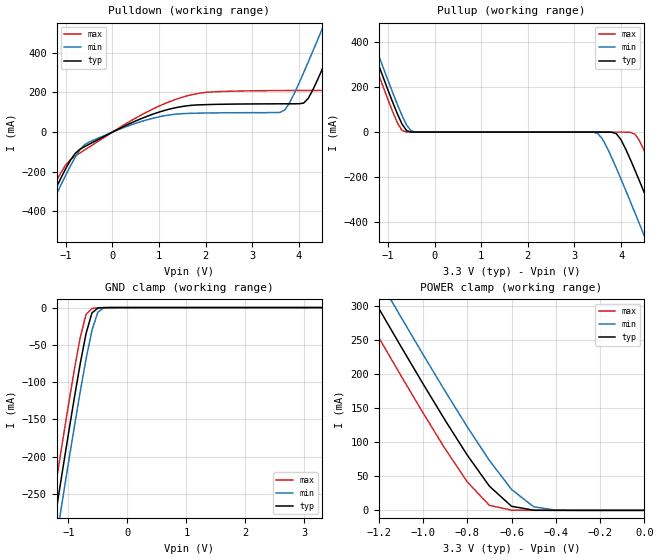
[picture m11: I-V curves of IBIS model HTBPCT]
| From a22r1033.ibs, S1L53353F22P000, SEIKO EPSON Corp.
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[Model]   HTBPCT
Model_type   Output
Polarity   Non-Inverting
|   typ   min   max
C_comp   5.0pF   4.0pF   6.0pF
|   typ   min   max
[Voltage range]   3.3   3.0   3.6
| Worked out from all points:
|   slope of the pulldown table from 0 to 0.495 V, typ, clamps not added: 8.88 ohm
|   GND clamp passes 1 mA (typ) near -0.51 V on its own axis
|   POWER clamp passes 1 mA (typ) near -0.51 V on its own axis
[Pulldown]
|   Voltage   I(typ)   I(min)   I(max)
-3.3V     -1.365A    -1.401A    -1.33A
-1.7V     -529.5mA   -566.9mA   -493.2mA
-1.1V     -229.2mA   -264.4mA   -201.9mA
-800mV    -107.9mA   -126.6mA   -121mA
200mV     23.74mA    19.01mA    29.63mA
1.7V      135.1mA    94.74mA    188.4mA
3.7V      142.6mA    112.5mA    209.5mA
4.1V      146mA      298.6mA    209.8mA
4.5V      316.8mA    521mA      210.2mA
4.9V      540.2mA    749.4mA    339.3mA
5.3V      769.7mA    980.3mA    562.8mA
6.6V      1.527A     1.738A     1.318A
[Pullup]
|   Voltage   I(typ)   I(min)   I(max)
-3.3V     1.514A     1.553A     1.476A
-1.6V     524.3mA    566.8mA    482.3mA
-1.5V     467mA      509.6mA    424.7mA
-800mV    81.11mA    122.6mA    41.82mA
-600mV    5.969mA    30.7mA     281.7uA
3.5V      -273.4nA   -6.157mA   -6.736nA
3.9V      -7.117mA   -160.6mA   -899.7nA
4.3V      -170mA     -359.4mA   -9.189mA
4.5V      -269.6mA   -461.5mA   -84mA
4.9V      -474.2mA   -667.8mA   -281.6mA
5.3V      -681.8mA   -875.9mA   -487.9mA
6.6V      -1.364A    -1.557A    -1.17A
[GND_clamp]
|   Voltage   I(typ)   I(min)   I(max)
-3.3V     -1.364A    -1.4A      -1.329A
-1.3V     -320.3mA   -359.4mA   -281.6mA
-1.2V     -269.6mA   -308.9mA   -230.8mA
-1.1V     -219.5mA   -258.7mA   -180.6mA
-1V       -170.1mA   -209.2mA   -131.4mA
-900mV    -121.9mA   -160.6mA   -84mA
-800mV    -75.86mA   -113.5mA   -40.55mA
-700mV    -34.75mA   -69.08mA   -9.194mA
-600mV    -7.118mA   -30.46mA   -1.232mA
-500mV    -657.9uA   -6.157mA   -258.3uA
-400mV    -61.96uA   -470.6uA   -20.17uA
3.3V      8.542nA    15.7uA     7.344nA
[POWER_clamp]
|   Voltage   I(typ)   I(min)   I(max)
-3.3V     1.514A     1.553A     1.476A
-1.3V     353.1mA    396.1mA    310.4mA
-1.2V     296.7mA    339.9mA    253.9mA
-1.1V     240.9mA    284.1mA    198mA
-1V       185.9mA    229mA      143.2mA
-900mV    132.3mA    175mA      90.33mA
-800mV    81.11mA    122.6mA    41.82mA
-700mV    35.52mA    73.27mA    7.314mA
-600mV    5.969mA    30.7mA     281.7uA
-500mV    284.1uA    5.285mA    30.01uA
-400mV    15.7uA     326.5uA    2.386uA
0V        8.542nA    18.22nA    8.664nA
[Ramp]
|   V_typ   V_min   V_max
dV/dt_r   1.98/0.68n   1.80/0.96n   2.16/0.47n
dV/dt_f   1.98/0.41n   1.80/0.55n   2.16/0.27n
R_load = 5000
